{attribute 'reflection'}
{attribute 'hide_all_locals'}
FUNCTION_BLOCK FB_EdgeCases EXTENDS FB_Base IMPLEMENTS I_Device
VAR_INPUT
    {attribute 'OPC.UA.DA' := '1'}
    fSetpoint : REAL := 0.0;
    sDescription : STRING(255) := 'Default description';
END_VAR
VAR_OUTPUT
    {attribute 'OPC.UA.DA.Access' := '1'}
    fActualValue : REAL;
END_VAR
VAR CONSTANT
    C_MAX_VALUE : REAL := 100.0;
    C_MIN_VALUE : REAL := -100.0;
END_VAR
VAR
    // Single line comment
    _state : INT;
    (* Block comment *)
    _timer : TON;
    (*
        Multi-line
        block comment
    *)
    _lastValue : REAL;
END_VAR

// Edge case: IF-ELSIF-ELSE chain
IF fSetpoint > C_MAX_VALUE THEN
    fActualValue := C_MAX_VALUE;
ELSIF fSetpoint < C_MIN_VALUE THEN
    fActualValue := C_MIN_VALUE;
ELSIF fSetpoint = 0.0 THEN
    fActualValue := _lastValue;
ELSE
    fActualValue := fSetpoint;
END_IF

// Edge case: Nested IF
IF _state = 1 THEN
    IF fSetpoint > 0.0 THEN
        IF _timer.Q THEN
            fActualValue := fSetpoint;
        END_IF
    END_IF
END_IF

// Edge case: WHILE loop
WHILE _state = 0 DO
    _state := 1;
END_WHILE

// Edge case: REPEAT-UNTIL
REPEAT
    _lastValue := fActualValue;
UNTIL _state <> 1
END_REPEAT

_lastValue := fActualValue;

METHOD PUBLIC FB_init : BOOL
VAR_INPUT
    bInitRetains : BOOL;
    bInCopyCode : BOOL;
END_VAR
_state := 0;
FB_init := TRUE;
END_METHOD

{attribute 'TcRpcEnable'}
METHOD ProcessData : BOOL
VAR_INPUT
    nSize : UDINT;
END_VAR
VAR
    i : UDINT;
END_VAR
FOR i := 0 TO nSize - 1 DO
    // Process each item
    _lastValue := _lastValue + 1.0;
END_FOR
ProcessData := TRUE;
END_METHOD

END_FUNCTION_BLOCK
